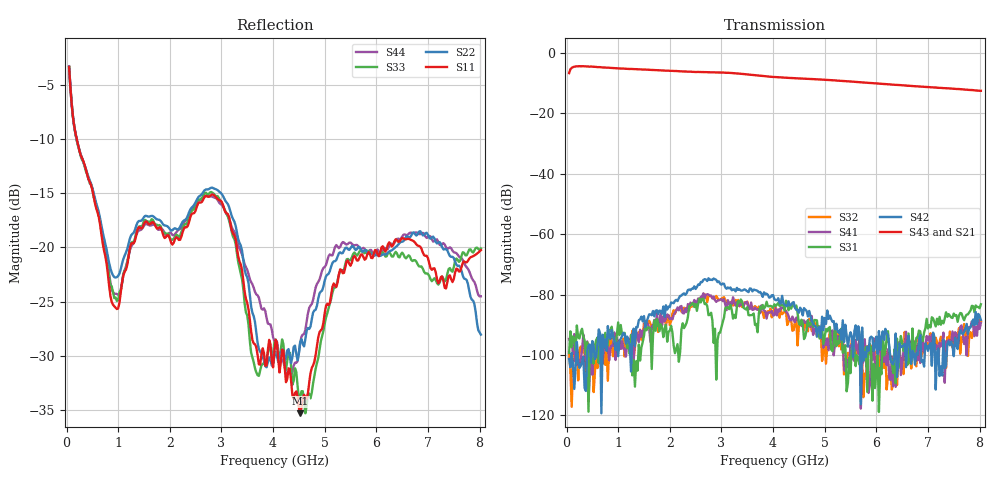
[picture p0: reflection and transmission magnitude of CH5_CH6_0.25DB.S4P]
!Agilent Technologies,E5071C,MY46316741,A.11.02
!Date: Mon Jun 01 10:39:16 2026
!Data & Calibration Information:
!1:CH5 INPUT 2:CH5 OUTPUT 3:CH6 INPUT 4:CH6 OUTPUT
!Freq	S11:SOLT4(ON)	S12:SOLT4(ON)	S13:SOLT4(ON)	S14:SOLT4(ON)
!	S21:SOLT4(ON)	S22:SOLT4(ON)	S23:SOLT4(ON)	S24:SOLT4(ON)
!	S31:SOLT4(ON)	S32:SOLT4(ON)	S33:SOLT4(ON)	S34:SOLT4(ON)
!	S41:SOLT4(ON)	S42:SOLT4(ON)	S43:SOLT4(ON)	S44:SOLT4(ON)
!PortZ  Port1:50+j0  Port2:50+j0  Port3:50+j0  Port4:50+j0
!Above PortZ is port z conversion or system Z0 setting when saving the data.
!When reading, reference impedance value at option line is always used.
# Hz S dB R 50
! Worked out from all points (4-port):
!   320 points, 50 MHz to 8.025 GHz, reference 50 ohm
!   strongest paths, dB at 50 MHz, 2.05 GHz, 4.05 GHz, 6.05 GHz, 8.025 GHz:
!     S43: -6.7, -6.0, -8.0, -10.2, -12.5
!     S21: -6.8, -6.1, -8.2, -10.4, -12.9
!     S42: -101.3, -82.7, -81.9, -92.1, -88.4
!     S31: -99.3, -92.5, -83.8, -118.9, -83.2
!     S41: -94.7, -88.2, -84.6, -97.0, -89.5
!     S32: -99.1, -86.5, -84.2, -100.6, -88.8
!   lowest |S11| = -35.3 dB at 4.525 GHz (marker M1), VSWR 1.04, Z = 49.5 - j1.65 ohm
!   |S11| at or under -10 dB: 197.6 MHz to end of sweep
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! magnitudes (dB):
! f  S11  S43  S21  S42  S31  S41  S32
! 50 MHz  -3.4  -6.7  -6.8  -101.3  -99.3  -94.7  -99.1
! 925 MHz  -25.4  -5.0  -5.2  -94.9  -95.2  -92.6  -93.2
! 2.85 GHz  -15.2  -6.4  -6.6  -74.7  -96.0  -80.7  -81.3
! 3.85 GHz  -30.9  -7.7  -7.9  -79.9  -84.0  -85.6  -85.5
! 4.525 GHz  -35.3  -8.5  -8.7  -84.3  -90.1  -89.2  -89.5
! 5.425 GHz  -21.3  -9.4  -9.6  -93.5  -112.0  -101.4  -103.5
! 8.025 GHz  -20.2  -12.5  -12.9  -88.4  -83.2  -89.5  -88.8
